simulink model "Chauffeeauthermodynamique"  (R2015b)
settings: Solver=ode15s  StartTime=0.0  StopTime=60000  RelTol=1e-3
libraries: fl_lib x9, nesl_utility x6

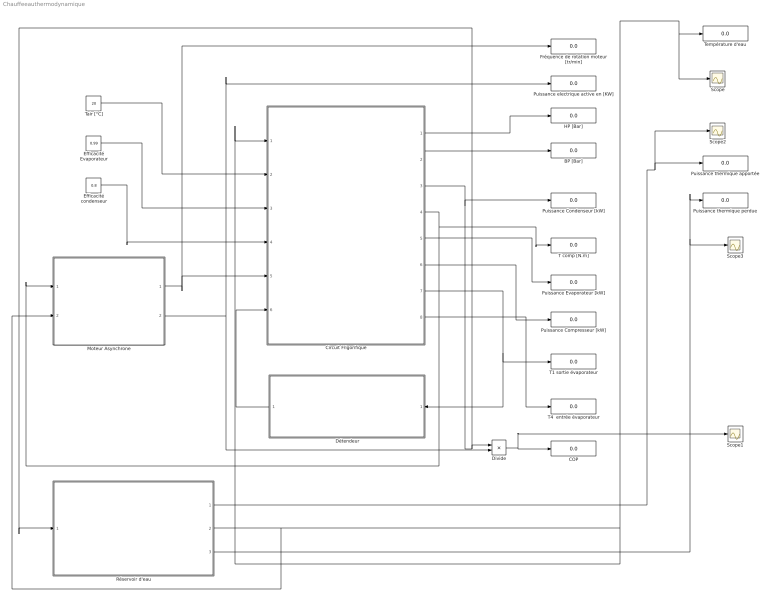
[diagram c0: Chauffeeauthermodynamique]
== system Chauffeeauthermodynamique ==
  BP [Bar] : Display
  COP : Display
  Circuit Frigorifique : Subsystem
  Divide : Product  Inputs=*/
  Détendeur : Subsystem
  Efficacité Evaporateur : Constant  Value=0.99
  Efficacité condenseur : Constant  Value=0.8
  Fréquence de rotation moteur [tr/min] : Display
  HP [Bar] : Display
  Moteur Asynchrone : Subsystem
  Puissance Compresseur [kW] : Display
  Puissance Condenseur [kW] : Display
  Puissance Evaporateur [kW] : Display
  Puissance electrique active en [KW] : Display
  Puissance thermique apportée : Display
  Puissance thermique perdue : Display
  Réservoir d'eau : Subsystem
  Scope{,1..3} (4 alike) : Scope
  T comp [N.m] : Display
  T1 sortie évaporateur : Display
  T4  entrée évaporateur : Display
  Tair [°C] : Constant  Value=20
  Température d'eau : Display
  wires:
  Efficacité Evaporateur/1 -> Circuit Frigorifique/3(Eff Evapo)
  Circuit Frigorifique/1(HP [bar]) -> HP [Bar]/1
  Circuit Frigorifique/2(BP [bar]) -> BP [Bar]/1
  Circuit Frigorifique/4(Tm [N.m]) -> Moteur Asynchrone/1(Tm [N.m]), T comp [N.m]/1
  Circuit Frigorifique/8(T4 [°C]) -> T4  entrée évaporateur/1
  Circuit Frigorifique/7(T1 [°C]) -> Détendeur/1(T1), T1 sortie évaporateur/1
  Circuit Frigorifique/5(Pevapo [kW]) -> Puissance Evaporateur [kW]/1
  Divide/1 -> Scope1/1, COP/1
  Circuit Frigorifique/6(Pcomp [kW]) -> Puissance Compresseur [kW]/1
  Efficacité condenseur/1 -> Circuit Frigorifique/4(effc)
  Détendeur/1(BP [Bar]) -> Circuit Frigorifique/6(BP[Bar])
  Moteur Asynchrone/2(Puissance Electrique active [W]) -> Puissance electrique active en [KW]/1, Divide/2
  Moteur Asynchrone/1(N [tr/min]) -> Fréquence de rotation moteur [tr/min]/1, Circuit Frigorifique/5(N [tr/min])
  Tair [°C]/1 -> Circuit Frigorifique/2(Tair [°C])
  Circuit Frigorifique/3(Pcond [kW]) -> Réservoir d'eau/1(" Puissance Condenseur [kW]"), Divide/1, Puissance Condenseur [kW]/1
  Réservoir d'eau/2(Température du réservoir [°C]) -> Moteur Asynchrone/2(Teau [°C]), Scope/1, Température d'eau/1, Circuit Frigorifique/1(Tee [°C])
  Réservoir d'eau/1(Puissance Condenseur [W]) -> Scope2/1, Puissance thermique apportée/1
  Réservoir d'eau/3(Puissance thermique perdue [W]) -> Scope3/1, Puissance thermique perdue/1

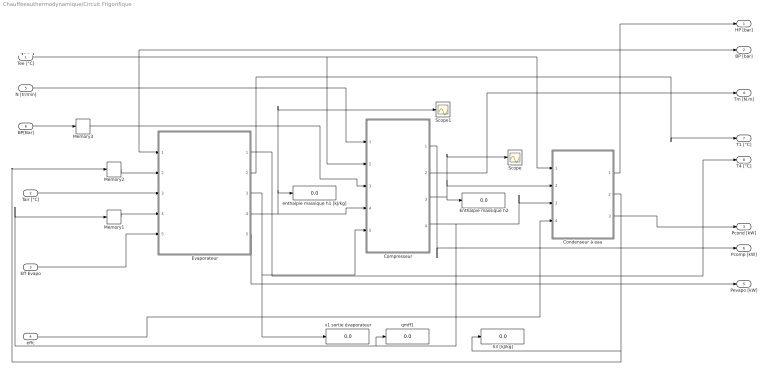
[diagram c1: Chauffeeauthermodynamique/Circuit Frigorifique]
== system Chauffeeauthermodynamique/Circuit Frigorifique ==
  note: +++++
  Tee [°C] : Inport
  Tair [°C] : Inport  Port=2
  Eff Evapo : Inport  Port=3
  effc : Inport  Port=4
  N [tr/min] : Inport  Port=5
  BP[Bar] : Inport  Port=6
  Compresseur : Subsystem
  Condenseur à eau : Subsystem
  Enthalpie massique h2 : Display
  Evaporateur : Subsystem
  Memory1 : Memory  X0=0.00001
  Memory2 : Memory  X0=300
  Memory3 : Memory  X0=2.5
  Scope : Scope
  Scope1 : Scope
  enthalpie massique h1 [kJ/kg] : Display
  h3 [kJ/kg] : Display
  qmff1 : Display
  v1 sortie évaporateur : Display
  HP [bar] : Outport
  BP [bar] : Outport  Port=2
  Pcond [kW] : Outport  Port=3
  Tm [N.m] : Outport  Port=4
  Pevapo [kW] : Outport  Port=5
  Pcomp [kW] : Outport  Port=6
  T1 [°C] : Outport  Port=7
  T4 [°C] : Outport  Port=8
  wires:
  Evaporateur/2(T1 [°C]) -> T1 [°C]/1
  N [tr/min]/1 -> Compresseur/1(N [tr/min])
  Evaporateur/5(Pévapo [kW]) -> Pevapo [kW]/1
  Tair [°C]/1 -> Evaporateur/3(Tair [°C])
  Memory1/1 -> Evaporateur/4(qmff [kg/s])
  Condenseur à eau/1(HP [bar]) -> HP [bar]/1
  BP[Bar]/1 -> Memory3/1
  Compresseur/4(qmff [kg/s]) -> Memory1/1, qmff1/1, Condenseur à eau/3(qmff [kg/s])
  Tee [°C]/1 -> Compresseur/2(Tee [°C]), Condenseur à eau/1(Tee [°C])
  Eff Evapo/1 -> Evaporateur/5(Eff)
  Evaporateur/3(v1 [m3/kg]) -> v1 sortie évaporateur/1, Compresseur/5(v1 [m3/kg])
  Condenseur à eau/2(h3 [kJ/kg]) -> Memory2/1, h3 [kJ/kg]/1
  Evaporateur/4(h1 [kJ/kg]) -> Compresseur/4(h1 [kJ/kg]), Scope1/1, enthalpie massique h1 [kJ/kg]/1
  Compresseur/3(h2 [kJ/kg]) -> Scope/1, Condenseur à eau/2(h2 [kJ/kg]), Enthalpie massique h2/1
  Compresseur/2(Tm [N.m]) -> Tm [N.m]/1
  Evaporateur/1(T4 [°C]) -> T4 [°C]/1
  Condenseur à eau/3(Pcond [kW]) -> Pcond [kW]/1
  Memory2/1 -> Evaporateur/2(h3 [kJ/kg])
  Compresseur/1(Pcomp [kW]) -> Pcomp [kW]/1
  effc/1 -> Condenseur à eau/4(effc)
  Memory3/1 -> BP [bar]/1, Compresseur/3(BP [bar]), Evaporateur/1(BP [bar])

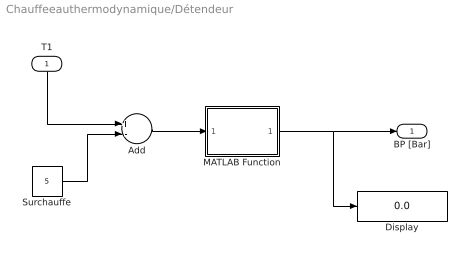
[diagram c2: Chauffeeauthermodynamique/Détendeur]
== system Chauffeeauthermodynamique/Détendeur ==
  T1 : Inport
  Add : Sum  Inputs=+-
  Display : Display
  MATLAB Function : MATLAB Function  TreatAsAtomicUnit=on
  Surchauffe : Constant  Value=5
  BP [Bar] : Outport
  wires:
  Add/1 -> MATLAB Function/1(T)
  T1/1 -> Add/1
  Surchauffe/1 -> Add/2
  MATLAB Function/1(BP) -> Display/1, BP [Bar]/1

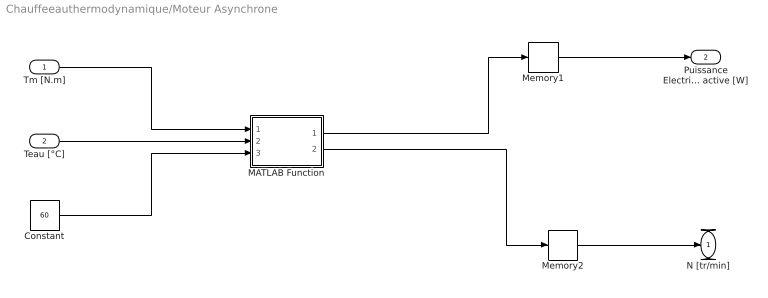
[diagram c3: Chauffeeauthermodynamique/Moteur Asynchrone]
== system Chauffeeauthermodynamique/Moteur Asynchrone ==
  Tm [N.m] : Inport
  Teau [°C] : Inport  Port=2
  Constant : Constant  Value=60
  MATLAB Function : MATLAB Function  TreatAsAtomicUnit=on
  Memory1 : Memory  X0=0.2
  Memory2 : Memory  X0=1480
  N [tr/min] : Outport
  Puissance Electrique active [W] : Outport  Port=2
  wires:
  Tm [N.m]/1 -> MATLAB Function/1(Tm)
  MATLAB Function/1(P) -> Memory1/1
  MATLAB Function/2(N) -> Memory2/1
  Memory1/1 -> Puissance Electrique active [W]/1
  Memory2/1 -> N [tr/min]/1
  Teau [°C]/1 -> MATLAB Function/2(Teau)
  Constant/1 -> MATLAB Function/3(Tcons)

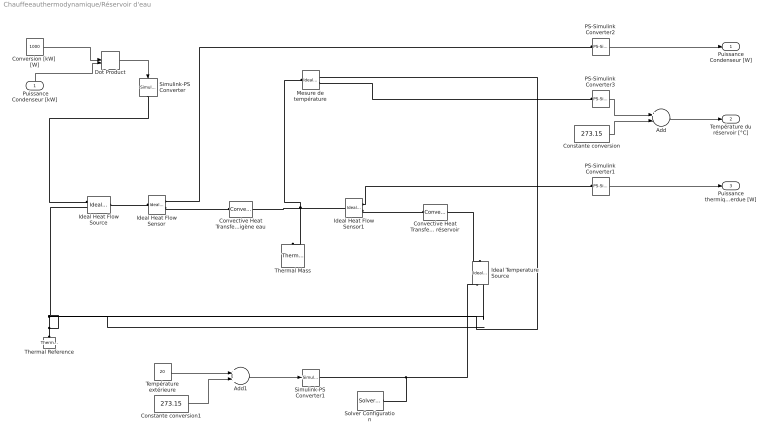
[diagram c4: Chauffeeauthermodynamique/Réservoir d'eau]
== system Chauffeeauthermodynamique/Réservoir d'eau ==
  " Puissance Condenseur [kW]" : Inport
  Add : Sum  Inputs=+-
  Add1 : Sum
  Constante conversion : Constant  Value=273.15
  Constante conversion1 : Constant  Value=273.15
  Convective Heat Transfer Echange Fluide frigorigène eau : fl_lib/Thermal/Thermal Elements/Convective Heat Transfer  area=0.82 m^2  heat_tr_coeff=25 W/(m^2 * K)  Q_specify=off  Q_priority=None  Q=0 J/s  T_specify=off  T_priority=None  T=0 K
  Convective Heat Transfer1 Echange avec l'extérieur du réservoir : fl_lib/Thermal/Thermal Elements/Convective Heat Transfer  area=1 m^2  heat_tr_coeff=0.0015 W/(m^2 * K)  Q_specify=off  Q_priority=None  Q=0 J/s  T_specify=off  T_priority=None  T=0 K
  Conversion [kW]  [W] : Constant  Value=1000
  Dot Product : DotProduct
  Ideal Heat Flow Sensor : fl_lib/Thermal/Thermal Sensors/Ideal Heat Flow Sensor
  Ideal Heat Flow Sensor1 : fl_lib/Thermal/Thermal Sensors/Ideal Heat Flow Sensor
  Ideal Heat Flow Source : fl_lib/Thermal/Thermal Sources/Ideal Heat Flow Source
  Ideal Temperature Source : fl_lib/Thermal/Thermal Sources/Ideal Temperature Source
  Mesure de température : fl_lib/Thermal/Thermal Sensors/Ideal Temperature Sensor
  PS-Simulink Converter1 : nesl_utility/PS-Simulink Converter  PhysicalDomain=network_engine_domain  SubClassName=ps_output  LeftPortType=input  RightPortType=output  PseudoPeriodic=off  Frequencies=[]  Unit=1  AffineConversion=off
  PS-Simulink Converter2 : nesl_utility/PS-Simulink Converter  PhysicalDomain=network_engine_domain  SubClassName=ps_output  LeftPortType=input  RightPortType=output  PseudoPeriodic=off  Frequencies=[]  Unit=1  AffineConversion=off
  PS-Simulink Converter3 : nesl_utility/PS-Simulink Converter  PhysicalDomain=network_engine_domain  SubClassName=ps_output  LeftPortType=input  RightPortType=output  PseudoPeriodic=off  Frequencies=[]  Unit=1  AffineConversion=off
  Simulink-PS Converter : nesl_utility/Simulink-PS Converter  PhysicalDomain=network_engine_domain  SubClassName=ps_input  LeftPortType=input  RightPortType=output  PseudoPeriodic=off  Frequencies=[]  NoiseDistribution=none  NoiseParameters=[]  Unit=1  AffineConversion=off  InputFiltering=off  SimscapeFilterOrder=1  InputFilterTimeConstant=.001  UdotUserProvided=1
  Simulink-PS Converter1 : nesl_utility/Simulink-PS Converter  PhysicalDomain=network_engine_domain  SubClassName=ps_input  LeftPortType=input  RightPortType=output  PseudoPeriodic=off  Frequencies=[]  NoiseDistribution=none  NoiseParameters=[]  Unit=K  AffineConversion=on  InputFiltering=off  SimscapeFilterOrder=1  InputFilterTimeConstant=.001  UdotUserProvided=1
  Solver Configuration : nesl_utility/Solver Configuration  PhysicalDomain=network_engine_domain  SubClassName=solver  LeftPortType=input  RightPortType=generic  Accelerate=off  Tones=[]  Harmonics=[]  SimulateNoise=off  Profile=off  UseLocalSampling=off  EnableSwitchedLinearOptims=on  FrequencyDomain=off  UseCCode=off  RelTol=0.001  AbsTol=1e-06  MinStep=1e-09  ToWorkspace=off  RevertToSquareIcSolve=off  NumHomotopyIterations=100  PhasorMode=off  PhasorModeNumHarmonics=1  DoDC=off  ResidualTolerance=1e-9  UseLocalSolver=off  LocalSolverChoice=NE_BACKWARD_EULER_ADVANCER  LocalSolverSampleTime=.001  DoFixedCost=off  MaxNonlinIter=3  MaxModeIter=2  LinearAlgebra=Sparse  DelaysMemoryBudget=1024  AutomaticFiltering=on  FilteringTimeConstant=0.001
  Température extérieure : Constant  Value=20
  Thermal Mass : fl_lib/Thermal/Thermal Elements/Thermal Mass  mass=200 kg  sp_heat=4185 J/kg/K  Q_specify=off  Q_priority=None  Q=0 J/s  T_specify=on  T_priority=High  T=15 C
  Thermal Reference : fl_lib/Thermal/Thermal Elements/Thermal Reference
  Puissance Condenseur [W] : Outport
  Température du réservoir [°C] : Outport  Port=2
  Puissance thermique perdue [W] : Outport  Port=3
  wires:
  " Puissance Condenseur [kW]"/1 -> Dot Product/2
  PS-Simulink Converter3/1 -> Add/1
  Add/1 -> Température du réservoir [°C]/1
  Constante conversion/1 -> Add/2
  Dot Product/1 -> Simulink-PS Converter/1
  Conversion [kW]  [W]/1 -> Dot Product/1
  PS-Simulink Converter1/1 -> Puissance thermique perdue [W]/1
  PS-Simulink Converter2/1 -> Puissance Condenseur [W]/1
  Add1/1 -> Simulink-PS Converter1/1
  Température extérieure/1 -> Add1/1
  Constante conversion1/1 -> Add1/2
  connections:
  Thermal Reference/LConn1 -- Ideal Temperature Source/RConn2 -- Mesure de température/RConn1 -- Ideal Heat Flow Source/RConn2
  Mesure de température/LConn1 -- Thermal Mass/LConn1 -- Ideal Heat Flow Sensor1/LConn1 -- Convective Heat Transfer Echange Fluide frigorigène eau/RConn1
  Solver Configuration/RConn1 -- Ideal Temperature Source/RConn1 -- Simulink-PS Converter1/RConn1
  Simulink-PS Converter/RConn1 -- Ideal Heat Flow Source/RConn1
  Convective Heat Transfer1 Echange avec l'extérieur du réservoir/RConn1 -- Ideal Temperature Source/LConn1
  PS-Simulink Converter3/LConn1 -- Mesure de température/RConn2
  Ideal Heat Flow Source/LConn1 -- Ideal Heat Flow Sensor/LConn1
  Ideal Heat Flow Sensor/RConn2 -- Convective Heat Transfer Echange Fluide frigorigène eau/LConn1
  Ideal Heat Flow Sensor1/RConn2 -- Convective Heat Transfer1 Echange avec l'extérieur du réservoir/LConn1
  Ideal Heat Flow Sensor1/RConn1 -- PS-Simulink Converter1/LConn1
  Ideal Heat Flow Sensor/RConn1 -- PS-Simulink Converter2/LConn1

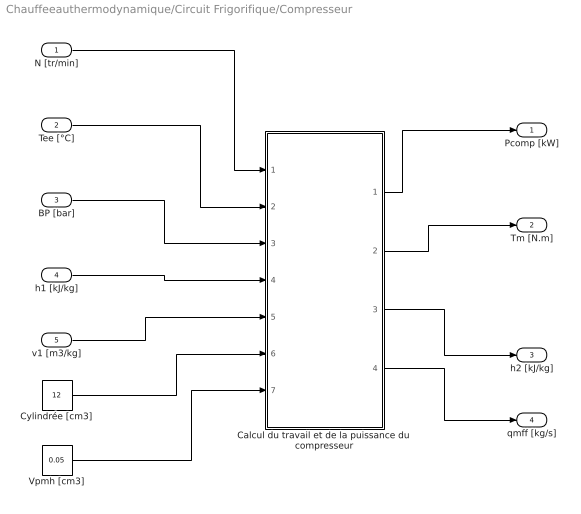
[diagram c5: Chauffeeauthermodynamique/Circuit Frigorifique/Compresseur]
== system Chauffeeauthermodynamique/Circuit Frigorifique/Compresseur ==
  N [tr/min] : Inport
  Tee [°C] : Inport  Port=2
  BP [bar] : Inport  Port=3
  h1 [kJ/kg] : Inport  Port=4
  v1 [m3/kg] : Inport  Port=5
  Calcul du travail et de la puissance du compresseur : MATLAB Function  TreatAsAtomicUnit=on
  Cylindrée [cm3] : Constant  Value=12
  Vpmh [cm3] : Constant  Value=0.05
  Pcomp [kW] : Outport
  Tm [N.m] : Outport  Port=2
  h2 [kJ/kg] : Outport  Port=3
  qmff [kg/s] : Outport  Port=4
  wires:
  Calcul du travail et de la puissance du compresseur/4(qmff) -> qmff [kg/s]/1
  Calcul du travail et de la puissance du compresseur/2(Tm) -> Tm [N.m]/1
  h1 [kJ/kg]/1 -> Calcul du travail et de la puissance du compresseur/4(h1)
  Tee [°C]/1 -> Calcul du travail et de la puissance du compresseur/2(Tee)
  BP [bar]/1 -> Calcul du travail et de la puissance du compresseur/3(BP)
  Calcul du travail et de la puissance du compresseur/1(P) -> Pcomp [kW]/1
  Calcul du travail et de la puissance du compresseur/3(h2) -> h2 [kJ/kg]/1
  N [tr/min]/1 -> Calcul du travail et de la puissance du compresseur/1(N)
  v1 [m3/kg]/1 -> Calcul du travail et de la puissance du compresseur/5(v1)
  Cylindrée [cm3]/1 -> Calcul du travail et de la puissance du compresseur/6(cyl)
  Vpmh [cm3]/1 -> Calcul du travail et de la puissance du compresseur/7(Vpmh)

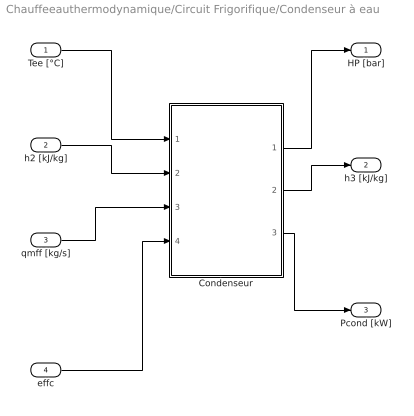
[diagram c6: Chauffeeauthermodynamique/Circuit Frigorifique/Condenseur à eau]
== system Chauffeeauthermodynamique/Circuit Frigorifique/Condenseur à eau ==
  Tee [°C] : Inport
  h2 [kJ/kg] : Inport  Port=2
  qmff [kg/s] : Inport  Port=3
  effc : Inport  Port=4
  Condenseur : MATLAB Function  TreatAsAtomicUnit=on
  HP [bar] : Outport
  h3 [kJ/kg] : Outport  Port=2
  Pcond [kW] : Outport  Port=3
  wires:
  Tee [°C]/1 -> Condenseur/1(Tee)
  Condenseur/1(HP) -> HP [bar]/1
  h2 [kJ/kg]/1 -> Condenseur/2(h2)
  qmff [kg/s]/1 -> Condenseur/3(qmff)
  Condenseur/2(h3) -> h3 [kJ/kg]/1
  Condenseur/3(Pcond) -> Pcond [kW]/1
  effc/1 -> Condenseur/4(eff)

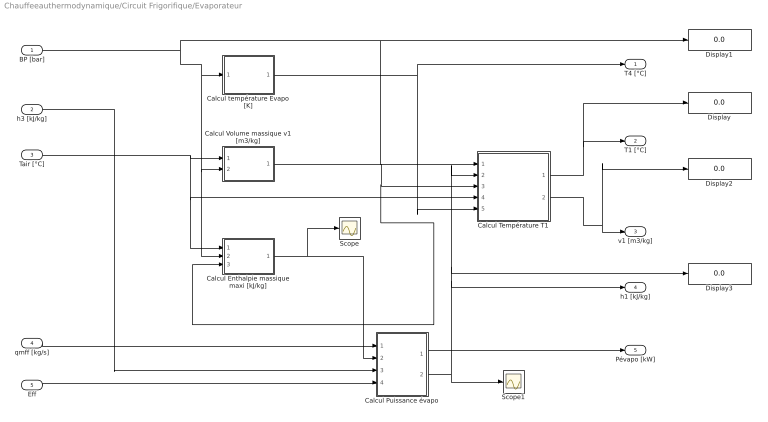
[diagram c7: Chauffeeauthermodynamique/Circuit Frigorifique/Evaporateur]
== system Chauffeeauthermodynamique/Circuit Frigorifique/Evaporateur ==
  BP [bar] : Inport
  h3 [kJ/kg] : Inport  Port=2
  Tair [°C] : Inport  Port=3
  qmff [kg/s] : Inport  Port=4
  Eff : Inport  Port=5
  Calcul Enthalpie massique maxi [kJ/kg] : MATLAB Function  TreatAsAtomicUnit=on
  Calcul Puissance évapo : MATLAB Function  TreatAsAtomicUnit=on
  Calcul Température T1 : MATLAB Function  TreatAsAtomicUnit=on
  Calcul Volume massique v1 [m3/kg] : MATLAB Function  TreatAsAtomicUnit=on
  Calcul température Evapo [K] : MATLAB Function  TreatAsAtomicUnit=on
  Display{,1..3} (4 alike) : Display
  Scope : Scope
  Scope1 : Scope
  T4 [°C] : Outport
  T1 [°C] : Outport  Port=2
  v1 [m3/kg] : Outport  Port=3
  h1 [kJ/kg] : Outport  Port=4
  Pévapo [kW] : Outport  Port=5
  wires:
  qmff [kg/s]/1 -> Calcul Puissance évapo/1(qmff)
  Calcul Enthalpie massique maxi [kJ/kg]/1(H) -> Scope/1, Calcul Puissance évapo/2(hmax)
  BP [bar]/1 -> Calcul Enthalpie massique maxi [kJ/kg]/2(P), Calcul Volume massique v1 [m3/kg]/2(P), Calcul température Evapo [K]/1(P), Display1/1, Calcul Température T1/1(P)
  Calcul température Evapo [K]/1(T) -> T4 [°C]/1, Calcul Température T1/5(T3)
  Tair [°C]/1 -> Calcul Enthalpie massique maxi [kJ/kg]/1(T), Calcul Température T1/4(T1max), Calcul Volume massique v1 [m3/kg]/1(T)
  Calcul Puissance évapo/1(Pevapo) -> Pévapo [kW]/1
  Eff/1 -> Calcul Puissance évapo/4(eff)
  Calcul Volume massique v1 [m3/kg]/1(v) -> Calcul Enthalpie massique maxi [kJ/kg]/3(v), Calcul Température T1/3(v)
  Calcul Température T1/2(v1) -> Display2/1, v1 [m3/kg]/1
  Calcul Température T1/1(T1) -> Display/1, T1 [°C]/1
  Calcul Puissance évapo/2(h1) -> h1 [kJ/kg]/1, Display3/1, Calcul Température T1/2(h), Scope1/1
  h3 [kJ/kg]/1 -> Calcul Puissance évapo/3(h3)

== matlab function Chauffeeauthermodynamique/Circuit Frigorifique/Compresseur/Calcul du travail
et de la puissance 
du compresseur ==
function [ P , Tm , h2 , qmff] = fcn( N , Tee , BP, h1 , v1 , cyl, Vpmh )
%#codegen

HP = 0.255 * Tee + 3.667 ;
if BP <0
BP = 1;
end
d1 = 2.49202E-01;
d2 = 2.45251E-03;
d3 = -1.65650E-06;
d4 = 8.91048E-10;
d5 = -6.96764E+00;

T = (372 + 240 )/2 ;
cp = d1 + d2 * T + d3 * T * T + d4 * T * T * T + d5 / T ;

R = 8.14892E-04 * 100;
gam = cp / (cp - R) ;

Vpmb = (cyl+Vpmh)/1000000;%( 3.14 * 0.03 ^2 ) / 4 * 0.024; 
Vpmh = Vpmh/1000000;%( 3.14 * 0.03 ^2 ) / 4 * 0.003;

HP = HP * 1e5;
BP = BP * 1e5;

Wtot = Vpmb * gam / ( gam - 1 ) * ( HP * ( HP / BP )^(- 1 / gam) -BP ) - Vpmh * ( HP - BP );

if N > 0
P = Wtot * N / 60 / 1000;
else
P = 0;
end

neff = 0.8 - 0.004 * (( HP / BP - 5 ) ^2 ) - 0.5 / ( HP / BP - 0.3 );
nv = 0.9 * ( 1 + Vpmh / ( Vpmb - Vpmh ) * ( 1 - ( HP / BP ) ^ 0.72 )); 

if N > 0
qmff = nv * (Vpmb - Vpmh) / v1 * N / 60;
else
    qmff = 0;
end

h2 = h1 + Wtot /1000 / nv /(Vpmb - Vpmh) * v1 ;


Tm = Wtot / neff / 2 / 3.14 ;


end

== matlab function Chauffeeauthermodynamique/Circuit Frigorifique/Evaporateur/Calcul Volume massique
 v1 [m3//kg] ==
function v = f134a(T,P)
%calcule la valeur du volume spécifique à partir de T et P
T = T + 273.15 ;
%if P < 1
%    P = 1;
%end
Tc = 374.21;
%Pc = 40.59;
R = 8.14892E-04;
e1 = -1.40114E-03;
e2 = 2.19433E-06;
e3 = -6.73580E-10;
e4 = -4.66800E-12;
f1 = 1.63714E-06;
f2 = -2.78860E-09;
f4 = 1.02574E-14;
g1 = -2.69555E-02;
g2 = 2.67772E-05;
g4 = 1.69513E-10;

b = 2.99628E-04;
k = 5.475;

Tr = T / Tc;
Zmax = 1;
Zmin = 0.008;
z = 0;    
    while Zmax - Zmin >= 0.00000001
    Zmoy = (Zmax + Zmin) / 2;
    z = Zmoy;
    zer = P - R * T / z - (e1 + f1 * T + g1 * exp(-k * Tr)) / (z * z) - (e2 + f2 * T + g2 * exp(-k * Tr)) / (z * z * z) - e3 / (z * z * z * z) - (e4 + f4 * T + g4 * exp(-k * Tr)) / (z * z * z * z * z);
    fzmoy = zer;
    z = Zmin;
    zer = P - R * T / z - (e1 + f1 * T + g1 * exp(-k * Tr)) / (z * z) - (e2 + f2 * T + g2 * exp(-k * Tr)) / (z * z * z) - e3 / (z * z * z * z) - (e4 + f4 * T + g4 * exp(-k * Tr)) / (z * z * z * z * z);
    fzmin = zer;

        if fzmoy * fzmin < 0
        Zmax = Zmoy;
        elseif fzmoy * fzmin > 0
        Zmin = Zmoy;
        end
        z = Zmoy;
        
    end
        
    v = z + b ;
    
end

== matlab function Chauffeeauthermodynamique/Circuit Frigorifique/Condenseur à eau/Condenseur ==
function [HP, h3 , Pcond] = fcn(Tee,h2,qmff,eff)
%#codegen
Tc = 374.21;

HP = 0.232 * Tee + 5.497 ;

Tr = (Tee + 273.15)/Tc;

h3max = 13807 * Tr ^5 - 50330* Tr^4 + 73272 * Tr^3 - 53050 * Tr ^2 + 19531* Tr - 2860;

h3 = h2 - (h2 - h3max)* eff;
if qmff >0
Pcond  = (h2 -h3)*qmff ;
else
   Pcond = 0;
end   


end

== matlab function Chauffeeauthermodynamique/Circuit Frigorifique/Evaporateur/Calcul température Evapo
[K] ==
function T = f134a(P)
% calcul de la BP à partir de la valeur de la température
if P < 1
    P = 1;
end
a1g = -7.7069E+00;
a2g = 2.4932E+00;
a3g = -2.9212E+00;
a4g = -3.8684E+00;
a5g = 4.6898E-01;
a6g = -8.3360E-05;
b1 = 1.5158;
b2 = 1.9907;
b3 = 4.3798;
b4 = 1.7461;
Tc = 374.21;
Pc = 40.59; 
Pr = P / Pc;

Tmax = Tc;
Tmin = 100;
Tmoy = 100;
while Tmax - Tmin >= 0.000000001
Tmoy = (Tmax + Tmin) / 2 ;
Tr = Tmoy / Tc;
zer = Pr - exp((a1g * (1 - Tr) + a2g * (1 - Tr) ^ b1 + a3g * (1 - Tr) ^ b2 + a4g * (1 - Tr) ^ b3 + a5g * (1 - Tr) ^ b4 + a6g) / Tr);
zermax = zer;
Tr = Tmin / Tc;
zer = Pr - exp((a1g * (1 - Tr) + a2g * (1 - Tr) ^ b1 + a3g * (1 - Tr) ^ b2 + a4g * (1 - Tr) ^ b3 + a5g * (1 - Tr) ^ b4 + a6g) / Tr);
zermin = zer;

if zermax * zermin < 0
    Tmax = Tmoy ;
elseif zermax * zermin > 0
    Tmin = Tmoy ;
end
Tmoy = (Tmax + Tmin) / 2 ;

end
    
       
T = Tmoy-273.15; %Tr * Tc;
end

== matlab function Chauffeeauthermodynamique/Circuit Frigorifique/Evaporateur/Calcul Enthalpie massique
 maxi [kJ//kg] ==
function H = f134a(T,P,v)
%calcule la valeur du volume spécifique à partir de T et P



Tc = 374.21;
Pc = 40.59;

R = 8.14892E-04;

d1 = 2.49202E-01;
d2 = 2.45251E-03;
d3 = -1.65650E-06;
%d4 = 8.91048E-10;
d5 = -6.96764E+00;

e1 = -1.40114E-03;
e2 = 2.19433E-06;
e3 = -6.73580E-10;
e4 = -4.66800E-12;

%f1 = 1.63714E-06;
%f2 = -2.78860E-09;
%f4 = 1.02574E-14;

g1 = -2.69555E-02;
g2 = 2.67772E-05;
g4 = 1.69513E-10;

b = 2.99628E-04;
k = 5.475;

Ho = 295.57 ;

z = v - b;
T = T + 273.15;
Tr = T / Tc ;

H = Ho + 100*(P * v - R * T) + d1 * T + d2 * T * T /2 + d3 * T * T * T / 3 + d5 * log(T) + 100* ( e1 / z + e2 / 2 / z / z + e3 / 3 / z / z / z + e4 / 4 / z / z / z / z + exp(-k*Tr)*(1+k*Tr) * ( g1 / z + g2 / 2 / z / z + g4 / 4 / z / z / z / z ));
if H > 500
    H = 500;
end
%H = d1 * T + d2 * T * T /2 + d3 * T * T * T / 3 + d5 * log(T);

    
end

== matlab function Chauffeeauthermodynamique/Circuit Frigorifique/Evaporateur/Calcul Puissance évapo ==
function [Pevapo,h1] = f134a(qmff,hmax,h3,eff)
%calcule la valeur du volume spécifique à partir de T et P
h1 = h3 + (hmax - h3 ) * eff ;
Pevapo = qmff * (hmax -h3) * eff;
    
end

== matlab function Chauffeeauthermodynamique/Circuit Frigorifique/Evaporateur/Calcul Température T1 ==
function [T1,v1] = f134a(P,h,v,T1max,T3)
%calcule la valeur du volume spécifique à partir de T et P

T1max = T1max + 273.15;
T3 = T3 + 273.15;
if P < 1
    P = 1;
end

R = 8.14892E-04;
Tc = 374.21;
Pc = 40.59;
d1 = 2.49202E-01;
d2 = 2.45251E-03;
d3 = -1.65650E-06;
%d4 = 8.91048E-10;
d5 = -6.96764E+00;

e1 = -1.40114E-03;
e2 = 2.19433E-06;
e3 = -6.73580E-10;
e4 = -4.66800E-12;

f1 = 1.63714E-06;
f2 = -2.78860E-09;
f4 = 1.02574E-14;

g1 = -2.69555E-02;
g2 = 2.67772E-05;
g4 = 1.69513E-10;

b = 2.99628E-04;
k = 5.475;

Ho = 295.57 ;

Tmax = T1max;
Tmin = T3 ;
T = 0;

while (Tmax - Tmin) >= 0.001
    
Tmoy = ( Tmax + Tmin ) / 2 ;

T = Tmoy;
Tr = T / Tc ;

Zmax = 1;
Zmin = 0.008;
z = 0;    
    while Zmax - Zmin >= 0.00000001
    Zmoy = (Zmax + Zmin) / 2;
    z = Zmoy;
    zer = P - R * T / z - (e1 + f1 * T + g1 * exp(-k * Tr)) / (z * z) - (e2 + f2 * T + g2 * exp(-k * Tr)) / (z * z * z) - e3 / (z * z * z * z) - (e4 + f4 * T + g4 * exp(-k * Tr)) / (z * z * z * z * z);
    fzmoy = zer;
    z = Zmin;
    zer = P - R * T / z - (e1 + f1 * T + g1 * exp(-k * Tr)) / (z * z) - (e2 + f2 * T + g2 * exp(-k * Tr)) / (z * z * z) - e3 / (z * z * z * z) - (e4 + f4 * T + g4 * exp(-k * Tr)) / (z * z * z * z * z);
    fzmin = zer;

        if fzmoy * fzmin < 0
        Zmax = Zmoy;
        elseif fzmoy * fzmin > 0
        Zmin = Zmoy;
        end
        z = Zmoy;
        
    end
        
    v = z + b ;
    
zerhmax = h - (Ho + 100*(P * v - R * T) + d1 * T + d2 * T * T /2 + d3 * T * T * T / 3 + d5 * log(T) + 100* ( e1 / z + e2 / 2 / z / z + e3 / 3 / z / z / z + e4 / 4 / z / z / z / z + exp(-k*Tr)*(1+k*Tr) * ( g1 / z + g2 / 2 / z / z + g4 / 4 / z / z / z / z )));

T = Tmin;
Tr = T / Tc ;

Zmax = 1;
Zmin = 0.008;
z = 0;    
    while Zmax - Zmin >= 0.00000001
    Zmoy = (Zmax + Zmin) / 2;
    z = Zmoy;
    zer = P - R * T / z - (e1 + f1 * T + g1 * exp(-k * Tr)) / (z * z) - (e2 + f2 * T + g2 * exp(-k * Tr)) / (z * z * z) - e3 / (z * z * z * z) - (e4 + f4 * T + g4 * exp(-k * Tr)) / (z * z * z * z * z);
    fzmoy = zer;
    z = Zmin;
    zer = P - R * T / z - (e1 + f1 * T + g1 * exp(-k * Tr)) / (z * z) - (e2 + f2 * T + g2 * exp(-k * Tr)) / (z * z * z) - e3 / (z * z * z * z) - (e4 + f4 * T + g4 * exp(-k * Tr)) / (z * z * z * z * z);
    fzmin = zer;

        if fzmoy * fzmin < 0
        Zmax = Zmoy;
        elseif fzmoy * fzmin > 0
        Zmin = Zmoy;
        end
        z = Zmoy;
        
    end
        
    v = z + b ;

zerhmin = h - (Ho + 100*(P * v - R * T) + d1 * T + d2 * T * T /2 + d3 * T * T * T / 3 + d5 * log(T) + 100* ( e1 / z + e2 / 2 / z / z + e3 / 3 / z / z / z + e4 / 4 / z / z / z / z + exp(-k*Tr)*(1+k*Tr) * ( g1 / z + g2 / 2 / z / z + g4 / 4 / z / z / z / z )));


     if zerhmax*zerhmin < 0
        Tmax = Tmoy;
        elseif zerhmax*zerhmin > 0
        Tmin = Tmoy;
     end
        
end
   T1 = T-273.15;
   v1 = v;
end

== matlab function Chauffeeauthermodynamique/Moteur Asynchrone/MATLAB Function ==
function [P,N] = fcn(Tm,Teau,Tcons)
%#codegen
if Teau < Tcons
N = 1496 - 12.96*Tm ;
P = 0.55*(Tm * N / 60 * 2 * 3.14 / (0.003*Tm^5 - 0.045*Tm^4 + 0.228*Tm^3 - 0.553*Tm^2 + 0.779*Tm + 0.02))/1000 ;
else
N = 0;
P = 0;
end
end

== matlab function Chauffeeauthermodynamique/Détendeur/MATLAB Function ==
function BP = f134a(T)
% calcul de la BP à partir de la valeur de la température
T= T + 273.15;
a1g = -7.7069E+00;
a2g = 2.4932E+00;
a3g = -2.9212E+00;
a4g = -3.8684E+00;
a5g = 4.6898E-01;
a6g = -8.3360E-05;
b1 = 1.5158;
b2 = 1.9907;
b3 = 4.3798;
b4 = 1.7461;
Tc = 374.21;
Pc = 40.59; 
Tr = T / Tc;
Pr = exp((a1g * (1 - Tr) + a2g * (1 - Tr) ^ b1 + a3g * (1 - Tr) ^ b2 + a4g * (1 - Tr) ^ b3 + a5g * (1 - Tr) ^ b4 + a6g) / Tr);
BP = Pr * Pc;


end
